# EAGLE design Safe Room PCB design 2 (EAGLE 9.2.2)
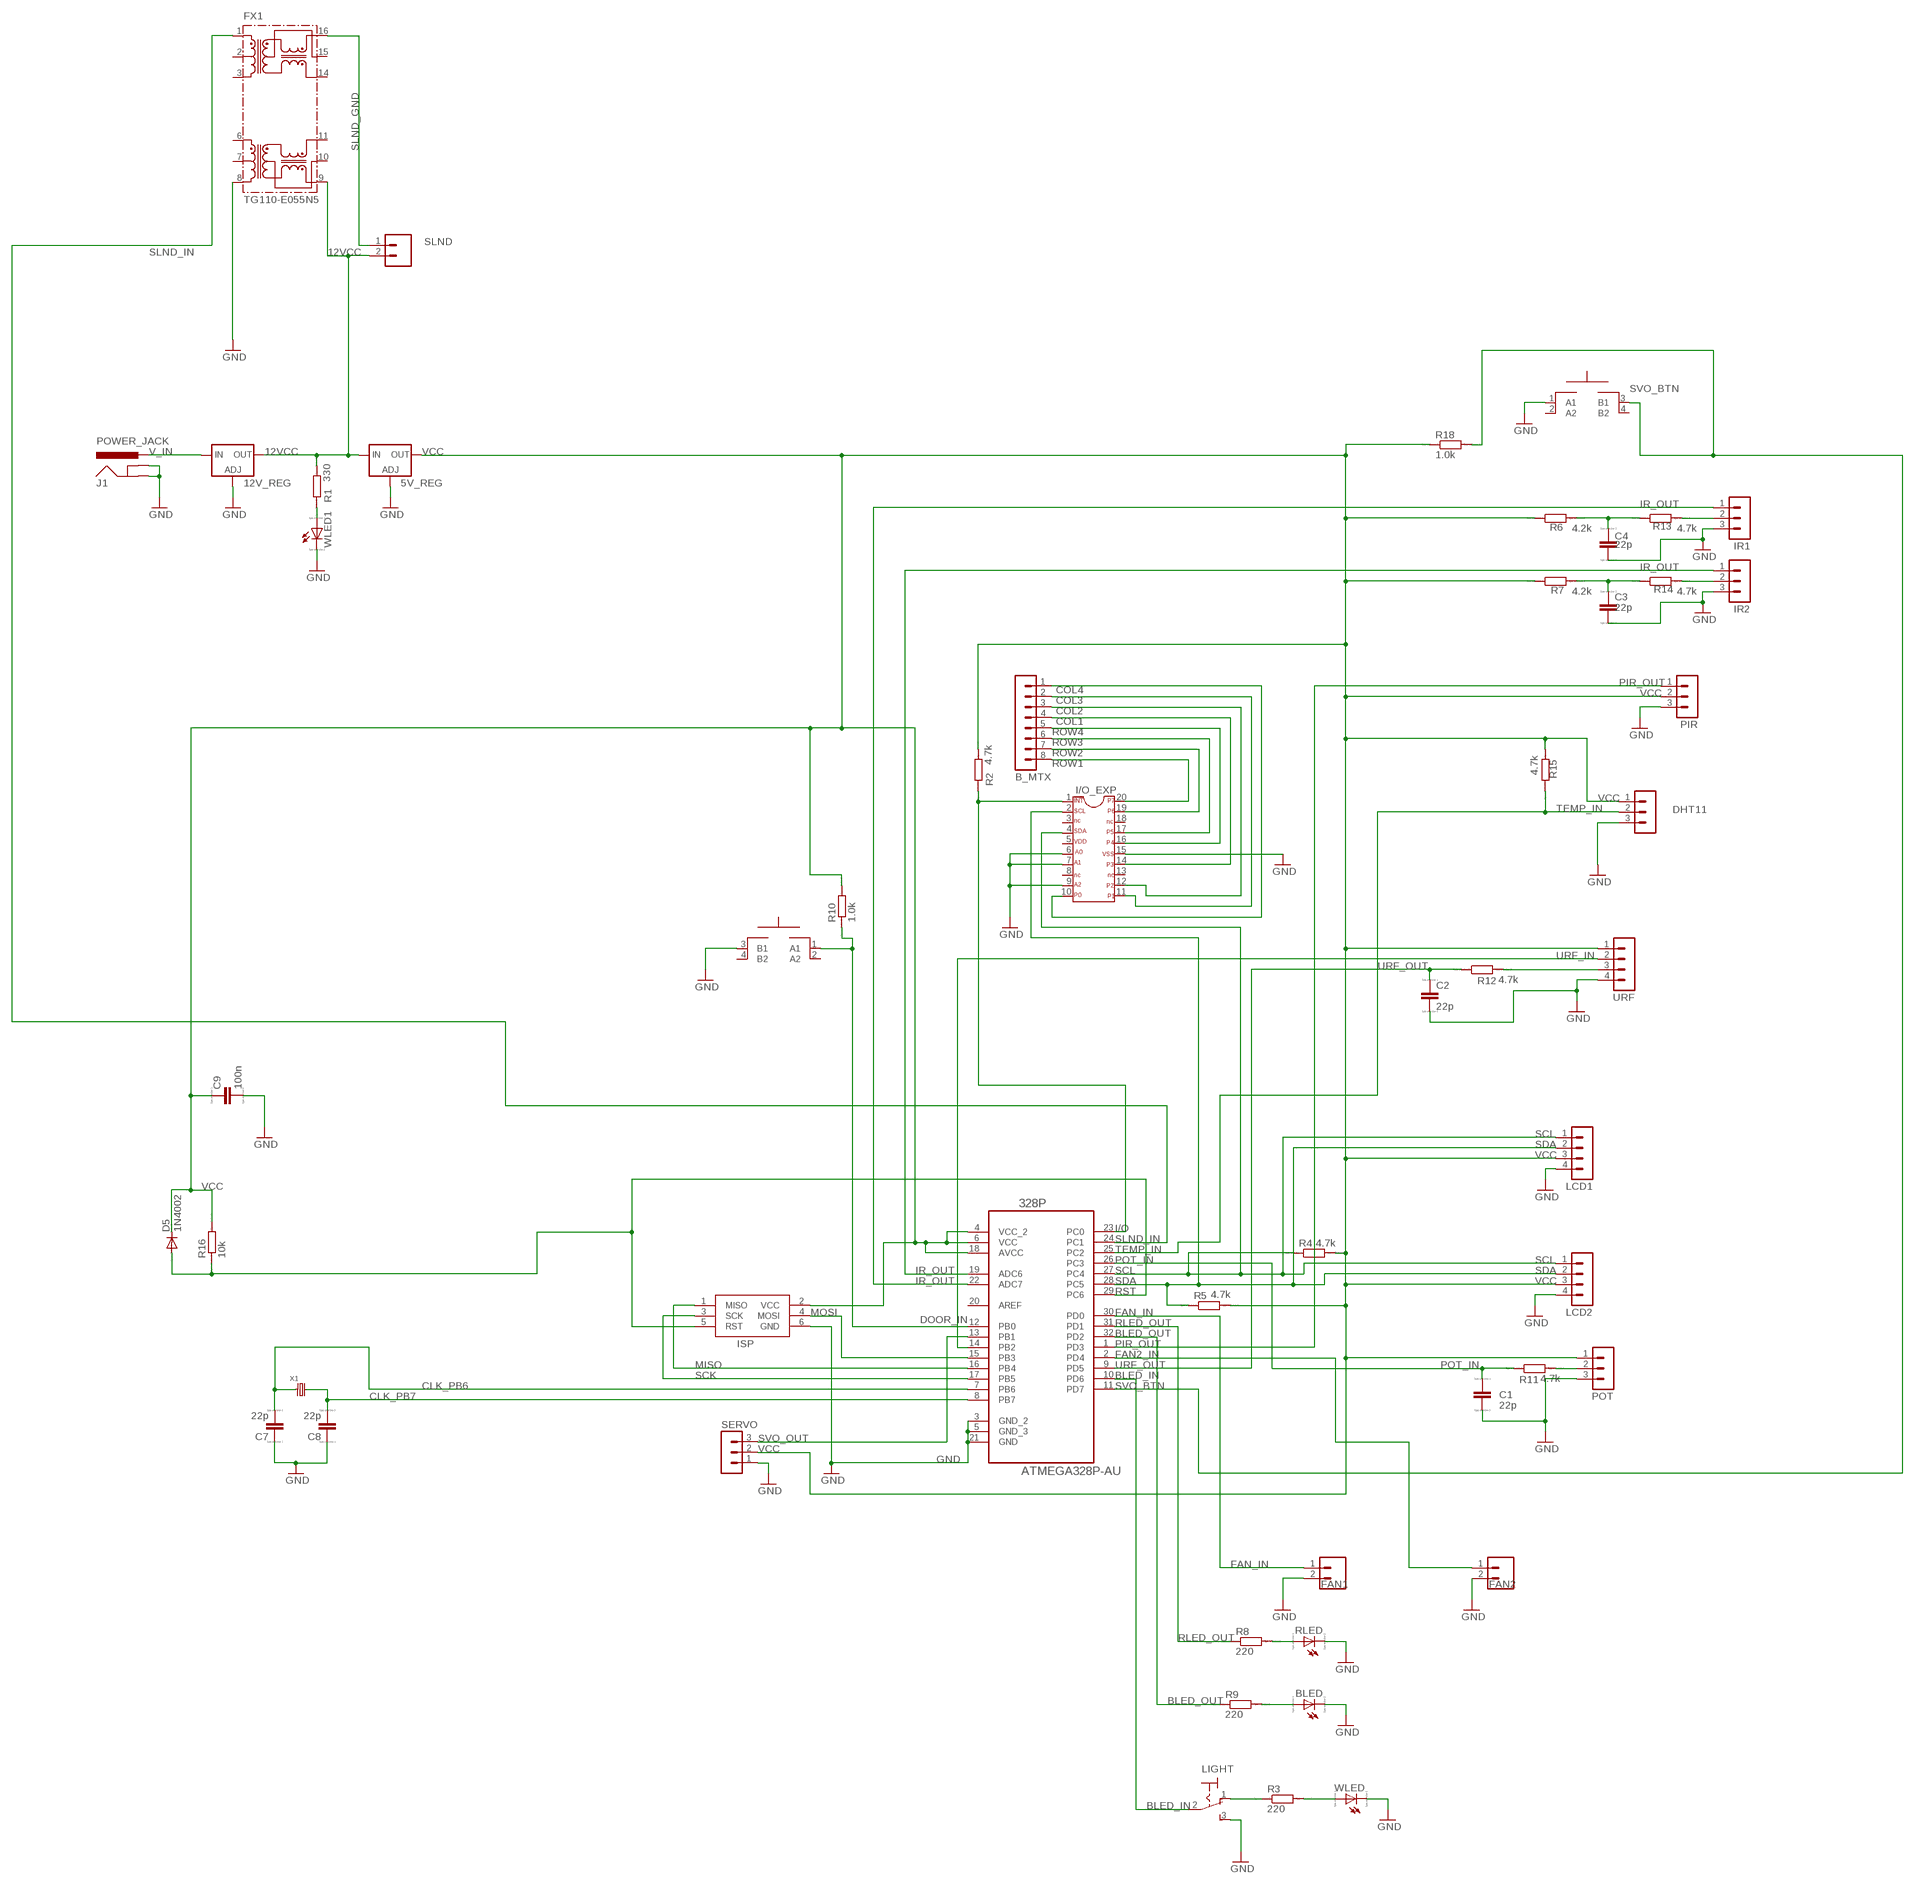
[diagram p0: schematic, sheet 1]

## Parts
5V_REG  LM317MBSTT3  [SOT223]
12V_REG  LD117AV50  [TO220L1]
328P  ATMEGA328P-AU  [QFP80P900X900X120-32N]
B_MTX  MA08-1  [MA08-1]
BLED  LED_E  [LED_1206]
C1  22p  C  [C0805]
C2  22p  C  [C0805]
C3  22p  C  [C0805]
C4  22p  C  [C0805]
C7  22p  C  [C0805]
C8  22p  C  [C0805]
C9  100n  C  [C0805]
D5  1N4002  1N4004  [DO41-10]
DHT11  MA03-1  [MA03-1]
DOOR  MOMENTARYBUTTON  [SPST_NO_SMD]
FAN1  M02  [02P]
FAN2  M02  [02P]
FX1  TG110-E055N5  [N5]
I/O_EXP  PCF8574_20TSSOP  [TSSOP20]
IR1  MA03-1  [MA03-1]
IR2  MA03-1  [MA03-1]
ISP  AVRISP-6  [AVRISP]
J1  POWER_JACK  [POWER_JACK_PTH]
LCD1  MA04-1  [MA04-1]
LCD2  MA04-1  [MA04-1]
LIGHT  320-916  [320-916]
PIR  MA03-1  [MA03-1]
POT  MA03-1  [MA03-1]
R1  330  R  [R0805]
R2  4.7k  R  [R0805]
R3  220  R  [R0805]
R4  4.7k  R  [R0805]
R5  4.7k  R  [R0805]
R6  4.2k  R  [R0805]
R7  4.2k  R  [R0805]
R8  220  R  [R0805]
R9  220  R  [R0805]
R10  1.0k  R  [R0805]
R11  4.7k  R  [R0805]
R12  4.7k  R  [R0805]
R13  4.7k  R  [R0805]
R14  4.7k  R  [R0805]
R15  4.7k  R  [R0805]
R16  10k  R  [R0805]
R18  1.0k  R  [R0805]
RLED  LED_E  [LED_1206]
SERVO  MA03-1  [MA03-1]
SLND  M02  [02P]
SVO_BTN  MOMENTARYBUTTON  [SPST_NO_SMD]
URF  MA04-1  [MA04-1]
WLED  LED_E  [LED_1206]
WLED1  LED_E  [LED_1206]
X1  ECS-80-18-5PX-TR  [HC49/US]

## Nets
12VCC: 5V_REG.3(IN) 12V_REG.2(OUT) FX1.9 R1.2 SLND.2
BLED_IN: 328P.10(PD6) LIGHT.2(P)
BLED_OUT: 328P.32(PD2) R9.1
CLK_PB6: 328P.7(PB6) C7.2 X1.P$1(XIN)
CLK_PB7: 328P.8(PB7) C8.2 X1.P$2(XOUT)
COL1: B_MTX.4 I/O_EXP.14
COL2: B_MTX.3 I/O_EXP.12
COL3: B_MTX.2 I/O_EXP.11
COL4: B_MTX.1 I/O_EXP.10
DOOR_IN: 328P.12(PB0) DOOR.1(A1) R10.1
FAN2_IN: 328P.2(PD4) FAN2.1
FAN_IN: 328P.30(PD0) FAN1.1
GND: 5V_REG.1(ADJ) 12V_REG.1(ADJ) 328P.3(GND_2) 328P.5(GND_3) 328P.21(GND) BLED.C C1.2 C2.2 C3.2 C4.2 C7.1 C8.1 C9.2 DHT11.3 DOOR.3(B1) FAN1.2 FAN2.2 FX1.8 I/O_EXP.6 I/O_EXP.7 I/O_EXP.9 I/O_EXP.15 IR1.3 IR2.3 ISP.6(GND) J1.GND J1.GNDBREAK LCD1.4 LCD2.4 LIGHT.3(S) PIR.3 POT.3 RLED.C SERVO.1 SVO_BTN.1(A1) URF.4 WLED1.C WLED.C
I/O: 328P.23(PC0) I/O_EXP.1 R2.1
IR_OUT: 328P.19(ADC6) 328P.22(ADC7) IR1.1 IR2.1
MISO: 328P.16(PB4) ISP.1(MISO)
MOSI: 328P.15(PB3) ISP.4(MOSI)
N$3: C3.1 R7.2 R14.1
N$4: R8.2 RLED.A
N$5: BLED.A R9.2
N$7: R3.2 WLED.A
N$8: R1.1 WLED1.A
N$9: LIGHT.1(O) R3.1
N$24: POT.2 R11.2
N$25: R12.2 URF.3
N$26: C4.1 R6.2 R13.1
N$27: IR2.2 R14.2
N$28: IR1.2 R13.2
PIR_OUT: 328P.1(PD3) PIR.1
POT_IN: 328P.26(PC3) C1.1 R11.1
RLED_OUT: 328P.31(PD1) R8.1
ROW1: B_MTX.8 I/O_EXP.20
ROW2: B_MTX.7 I/O_EXP.19
ROW3: B_MTX.6 I/O_EXP.17
ROW4: B_MTX.5 I/O_EXP.16
RST: 328P.29(PC6) D5.A ISP.5(RST) R16.1
SCK: 328P.17(PB5) ISP.3(SCK)
SCL: 328P.27(PC4) I/O_EXP.4 LCD1.1 LCD2.1 R4.1
SDA: 328P.28(PC5) I/O_EXP.2 LCD1.2 LCD2.2 R5.1
SLND_GND: FX1.16 SLND.1
SLND_IN: 328P.24(PC1) FX1.1
SVO_BTN: 328P.11(PD7) R18.2 SVO_BTN.3(B1)
SVO_OUT: 328P.13(PB1) SERVO.3
TEMP_IN: 328P.25(PC2) DHT11.2 R15.1
URF_IN: 328P.14(PB2) URF.2
URF_OUT: 328P.9(PD5) C2.1 R12.1
V_IN: 12V_REG.3(IN) J1.PWR
VCC: 5V_REG.4(OUT) 328P.4(VCC_2) 328P.6(VCC) 328P.18(AVCC) C9.1 D5.C DHT11.1 ISP.2(VCC) LCD1.3 LCD2.3 PIR.2 POT.1 R2.2 R4.2 R5.2 R6.1 R7.1 R10.2 R15.2 R16.2 R18.1 SERVO.2 URF.1
Unconnected: 328P.20(AREF) DOOR.2(A2) DOOR.4(B2) FX1.2 FX1.3 FX1.6 FX1.7 FX1.10 FX1.11 FX1.14 FX1.15 I/O_EXP.3 I/O_EXP.5 I/O_EXP.8 I/O_EXP.13 I/O_EXP.18 SVO_BTN.2(A2) SVO_BTN.4(B2)

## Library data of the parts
5V_REG = v-reg:LM317?*: 500 mA Adjustable Output Positive Voltage Regulator Source: http://www.onsemi.co.jp .. LM317M-D.PDF; PARTNUMBER: LM317M
12V_REG = ECE388:LD117A?*: Low drop fixed and adjustable positive voltage regulators 1 A Source: http://www.st.com/stonline/products/literature/ds/7194/ld1117axx.pdf
328P = Atmel_By_element14_Batch_1-00:ATMEGA328P-AU: 8-bit Microcontroller with In-System Programmable Flash; MPN: ATMEGA328P-AU; OC_FARNELL: 1715486; OC_NEWARK: 14R4631; PACKAGE: TQFP-32; SUPPLIER: Atmel
B_MTX = con-lstb:MA08-1: PIN HEADER; OC_FARNELL: unknown; OC_NEWARK: unknown
BLED RLED WLED WLED1 = eagle-ltspice:LED_E: LED; SPICEMODEL: NONE; SPICEPREFIX: D; SPICETYPE: diode
C1-C4 C7-C9 = eagle-ltspice:C: CAPACITOR, European symbol; SPICEMODEL: NONE; SPICEPREFIX: C
D5 = diode:1N4004: DIODE
DHT11 IR1 IR2 PIR POT SERVO = con-lstb:MA03-1: PIN HEADER; OC_FARNELL: unknown; OC_NEWARK: unknown
DOOR SVO_BTN = ECE388:MOMENTARYBUTTON
FAN1 FAN2 SLND = con-amp-quick:M02: AMP QUICK CONNECTOR; OC_FARNELL: unknown; OC_NEWARK: unknown
FX1 = halo-electronics:TG110-E*N5: E-Ultra (TM) 10/100BASE-TX SOIC-16 Fast Ethernet Magnetic Modules Source: www.haloelectronics.com .. e-ultra.pdf
I/O_EXP = MY_LIBRARY:PCF8574_20TSSOP
ISP = ECE388:AVRISP: AVR ISP HEADER Standard 6 pin header for AVR programming
J1 = SparkFun-Connectors:POWER_JACK: Power Jack Connector This is the standard 5.5mm barrel jack for power. The PTH is the most common, proven, reliable, footprint. The Slot footprint only works if the mill layer is transmitted to the PCB fab house so be warned. Here are the connectors we sell at SparkFun: DC Barrel Power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; PROD_ID: CONN-08197
LCD1 LCD2 URF = con-lstb:MA04-1: PIN HEADER; OC_FARNELL: unknown; OC_NEWARK: unknown
LIGHT = switch:320-916: TOGGLE SWITCH distributor RS Components
R1-R16 R18 = eagle-ltspice:R: RESISTOR, European symbol; SPICEMODEL: NONE; SPICEPREFIX: R
X1 = ECE388:ECS-80-18-5PX-TR

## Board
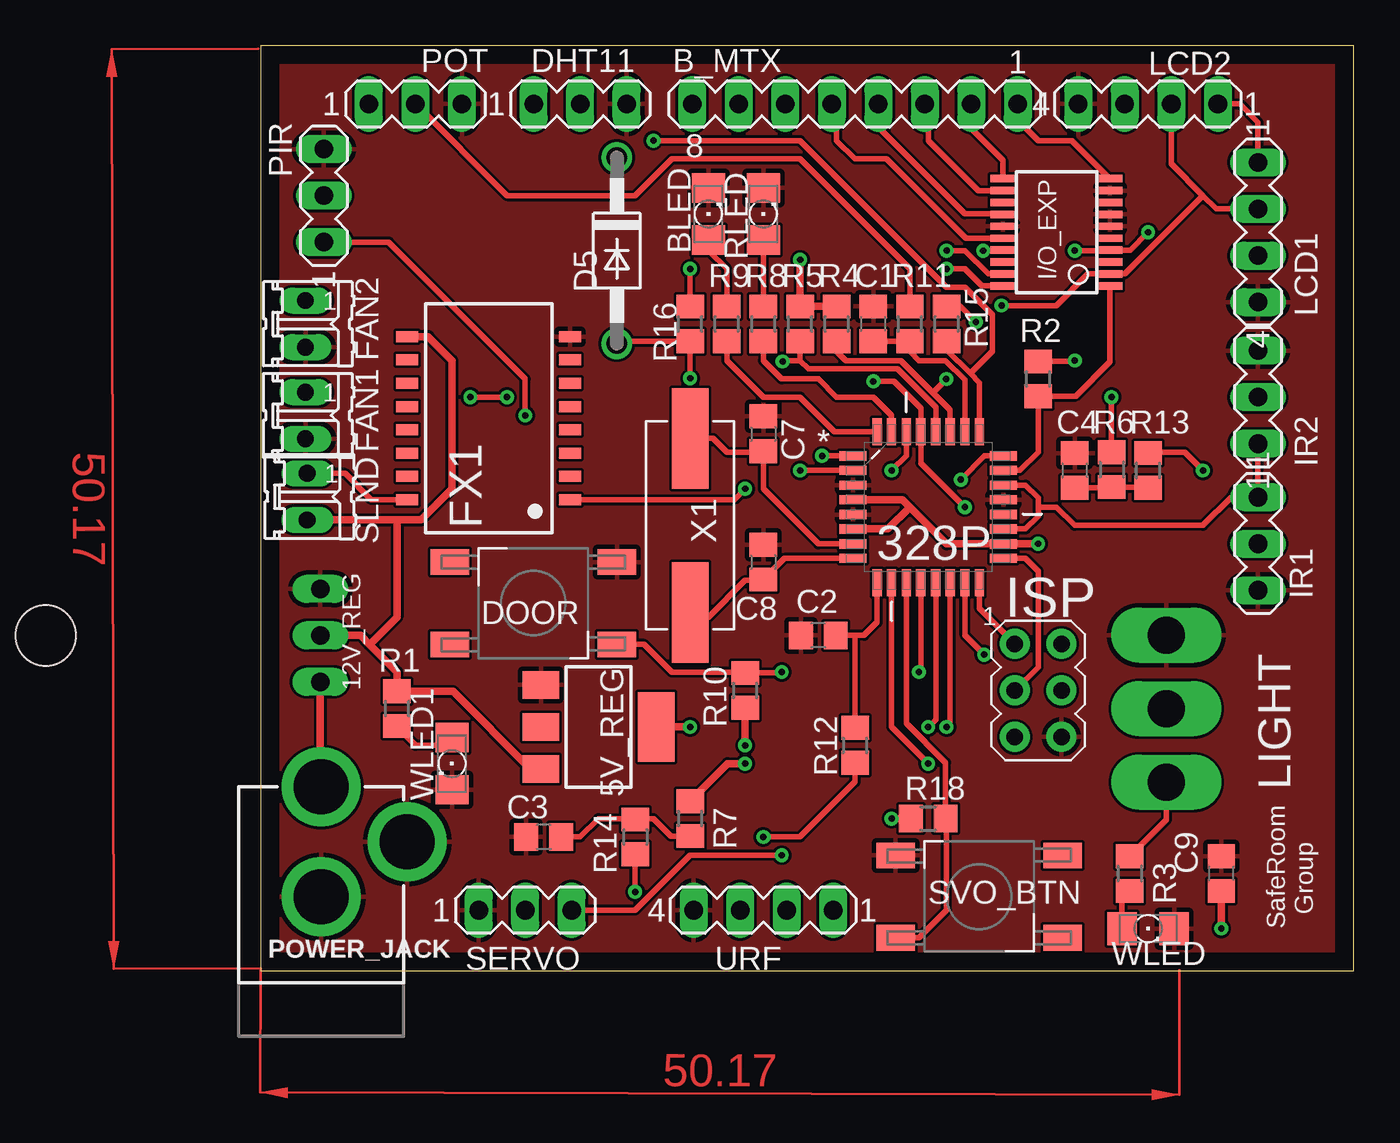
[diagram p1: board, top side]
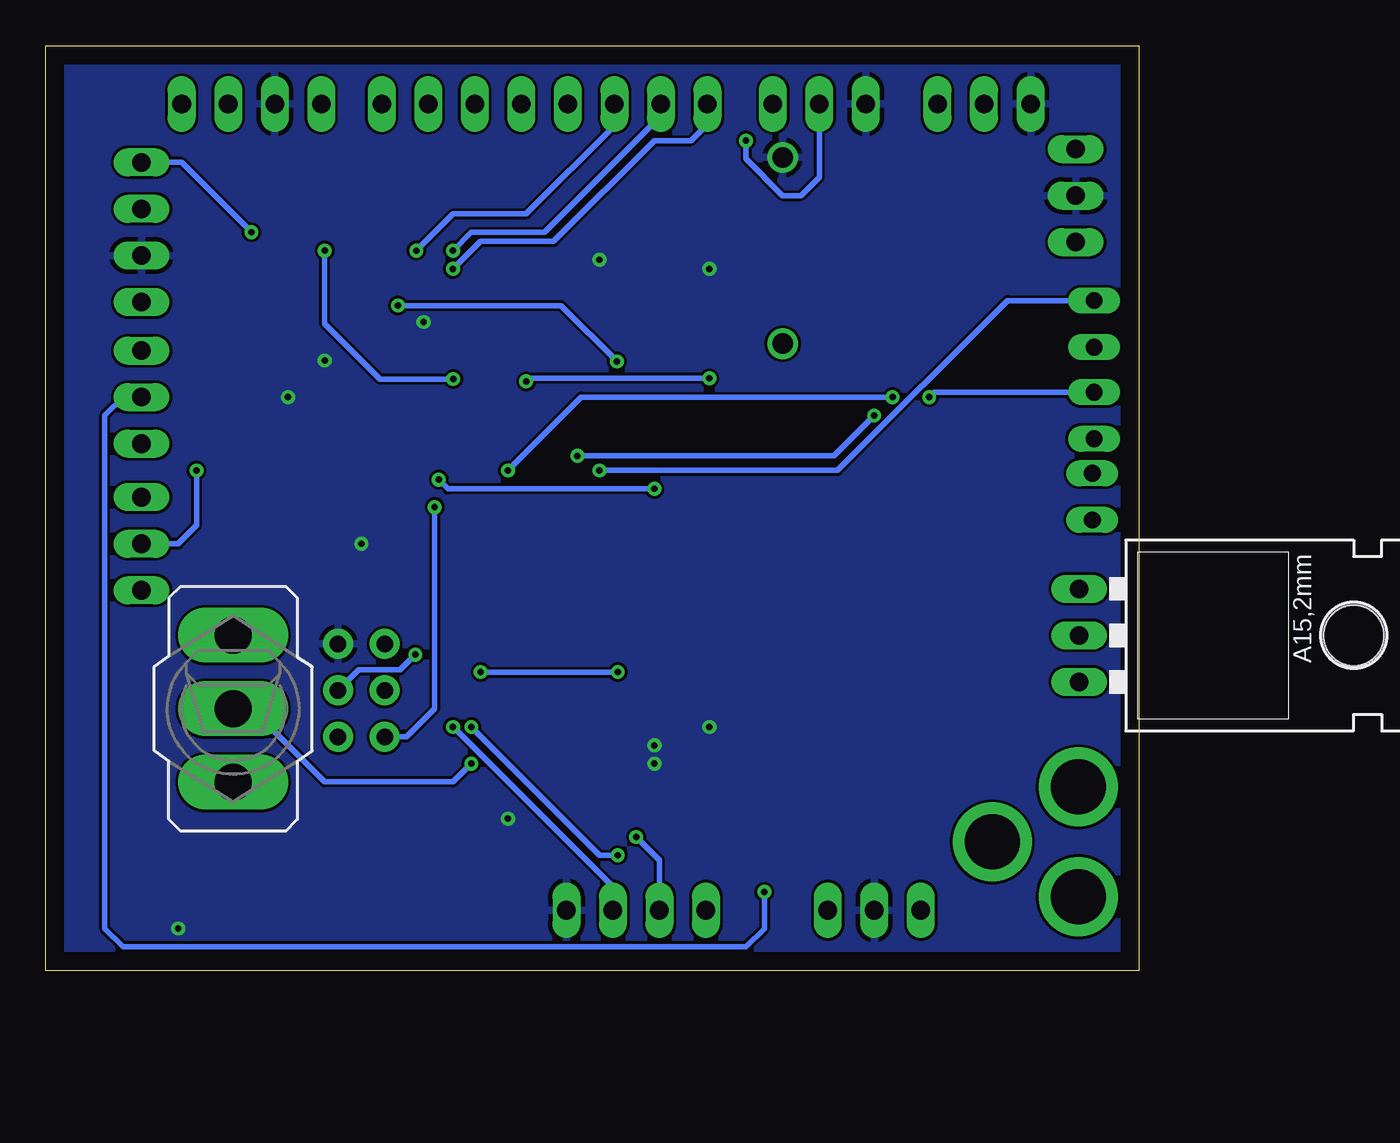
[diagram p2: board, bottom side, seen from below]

Size 59.67 x 50.48 mm. Coordinates in mm from the lower left corner, seen from the top.
Outline: 0,0 59.67,0 59.67,50.48 0,50.48 0,0
Copper layers (1*16): Top 0.035mm / dielectric 1.5mm / Bottom 0.035mm
Design rules "default": minimum track width 6mil, minimum drill 0.35mm, track to track 6mil, track to pad 6mil, pad to pad 6mil, via to via 6mil, smd to smd 6mil, copper to edge 40mil, drill to drill 6mil, minimum pad ring 10mil, minimum via ring 8mil, stop-mask expansion 4mil, vias tented up to drill 0mil, thermal gap 10mil

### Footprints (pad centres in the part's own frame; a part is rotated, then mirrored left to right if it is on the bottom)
SOT223 = smd 1.5 x 2: 1 -2.3,-3.15; 2 0,-3.15; 3 2.3,-3.15 | smd 3.8 x 2: 4 0,3.15
TO220L1 = drill 1.016 long: 1 -2.54,-3.81; 2 0,-3.81; 3 2.54,-3.81 | hole 3.302: 0,11.176
QFP80P900X900X120-32N = smd 1.473 x 0.508: 1 -4.115,2.794; 2 -4.115,2.007; 3 -4.115,1.194; 4 -4.115,0.406; 5 -4.115,-0.406; 6 -4.115,-1.194; 7 -4.115,-2.007; 8 -4.115,-2.794; 17 4.115,-2.794; 18 4.115,-2.007; 19 4.115,-1.194; 20 4.115,-0.406; 21 4.115,0.406; 22 4.115,1.194; 23 4.115,2.007; 24 4.115,2.794 | smd 0.508 x 1.473: 9 -2.794,-4.115; 10 -2.007,-4.115; 11 -1.194,-4.115; 12 -0.406,-4.115; 13 0.406,-4.115; 14 1.194,-4.115; 15 2.007,-4.115; 16 2.794,-4.115; 25 2.794,4.115; 26 2.007,4.115; 27 1.194,4.115; 28 0.406,4.115; 29 -0.406,4.115; 30 -1.194,4.115; 31 -2.007,4.115; 32 -2.794,4.115
MA08-1 = drill 1.016 long: 1 -8.89,0; 2 -6.35,0; 3 -3.81,0; 4 -1.27,0; 5 1.27,0; 6 3.81,0; 7 6.35,0; 8 8.89,0
LED_1206 = smd 1.6 x 1.803: A -1.422,0; C 1.422,0
C0805 = smd 1.3 x 1.5: 1 -0.95,0; 2 0.95,0
DO41-10 = drill 1.118: A 5.08,0; C -5.08,0
MA03-1 = drill 1.016 long: 1 -2.54,0; 2 0,0; 3 2.54,0
SPST_NO_SMD = smd 2.108 x 1.397: 1 0,4.496; 2 9.119,4.496; 3 0,0; 4 9.119,0
02P = drill 0.914 long: 1 -1.27,0; 2 1.27,0
N5 = smd 0.6 x 1.2: 1 -4.445,-4.445; 2 -3.175,-4.445; 3 -1.905,-4.445; 4 -0.635,-4.445; 5 0.635,-4.445; 6 1.905,-4.445; 7 3.175,-4.445; 8 4.445,-4.445; 9 4.445,4.445; 10 3.175,4.445; 11 1.905,4.445; 12 0.635,4.445; 13 -0.635,4.445; 14 -1.905,4.445; 15 -3.175,4.445; 16 -4.445,4.445
TSSOP20 = smd 0.4 x 1.35: 1 -2.925,-2.925; 2 -2.275,-2.925; 3 -1.625,-2.925; 4 -0.975,-2.925; 5 -0.325,-2.925; 6 0.325,-2.925; 7 0.975,-2.925; 8 1.625,-2.925; 9 2.275,-2.925; 10 2.925,-2.925; 11 2.925,2.925; 12 2.275,2.925; 13 1.625,2.925; 14 0.975,2.925; 15 0.325,2.925; 16 -0.325,2.925; 17 -0.975,2.925; 18 -1.625,2.925; 19 -2.275,2.925; 20 -2.925,2.925
AVRISP = drill 0.9 pad 1.626: 1 -1.27,2.54; 2 1.27,2.54; 3 -1.27,0; 4 1.27,0; 5 -1.27,-2.54; 6 1.27,-2.54
POWER_JACK_PTH = drill 2.997 pad 4.318: GND 0,7.7; GNDBREAK 4.7,10.7; PWR 0,13.7
MA04-1 = drill 1.016 long: 1 -3.81,0; 2 -1.27,0; 3 1.27,0; 4 3.81,0
320-916 = drill 2.007 long: 1 0,4.013; 2 0,0; 3 0,-4.013
R0805 = smd 1.3 x 1.5: 1 -0.95,0; 2 0.95,0
HC49/US = smd 5.5 x 2: P$1 -4.75,0; P$2 4.75,0

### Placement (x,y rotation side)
5V_REG  18.44,13.3 270 top
12V_REG  -0.56,18.3 270 bottom
328P  36.44,25.3 0 top
B_MTX  32.44,47.3 180 top
BLED  24.44,41.3 90 top
C1  33.44,35.3 90 top
C2  30.44,18.3 180 top
C3  15.44,7.3 180 top
C4  44.44,27.3 90 top
C7  27.44,29.3 270 top
C8  27.44,22.3 270 top
C9  52.44,5.3 90 top
D5  19.44,39.3 270 top
DHT11  17.44,47.3 0 top
DOOR  19.44,22.3 180 top
FAN1  2.44,30.3 270 top
FAN2  2.44,35.3 270 top
FX1  12.45,30.16 90 top
I/O_EXP  43.44,40.3 90 top
IR1  54.44,23.3 270 top
IR2  54.44,31.3 90 top
ISP  42.44,15.3 0 top
J1  3.3,-3.67 0 top
LCD1  54.44,40.3 270 top
LCD2  48.44,47.3 180 top
LIGHT  49.44,14.3 180 bottom
PIR  3.44,42.3 90 top
POT  8.44,47.3 0 top
R1  7.44,14.3 90 top
R2  42.44,32.3 90 top
R3  47.44,5.3 270 top
R4  31.44,35.3 90 top
R5  29.44,35.3 90 top
R6  46.46,27.35 270 top
R7  23.44,8.3 270 top
R8  27.44,35.3 90 top
R9  25.44,35.3 90 top
R10  26.44,15.3 270 top
R11  35.44,35.3 90 top
R12  32.44,12.3 270 top
R13  48.44,27.3 90 top
R14  20.44,7.3 270 top
R15  37.44,35.3 90 top
R16  23.44,35.3 90 top
R18  36.44,8.3 0 top
RLED  27.44,41.3 90 top
SERVO  14.44,3.3 0 top
SLND  2.54,25.88 270 top
SVO_BTN  34.67,1.8 0 top
URF  27.44,3.3 180 top
WLED  48.44,2.3 0 top
WLED1  10.44,11.3 270 top
X1  23.44,24.3 270 top

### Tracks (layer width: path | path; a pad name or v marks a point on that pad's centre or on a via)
12VCC
  Top 0.406: 5V_REG.3 14.74,11 10.49,15.25 R1.2 7.44,16.3 5.94,17.8 | 12V_REG.2 5.44,18.3 5.94,17.8 | SLND.2 7.44,24.61 | 7.44,24.61 8.75,24.61 10.44,26.3 10.44,33.3 9.14,34.6 FX1.9 | 7.44,24.61 7.44,19.3 5.94,17.8
BLED_IN  (via drill 0.35 pad 0.55)
  Top 0.305: 328P.10 34.44,13.31 v36.44,11.3
  Bottom 0.305: v36.44,11.3 37.44,10.3 44.44,10.3 48.44,14.3 LIGHT.2
BLED_OUT
  Top 0.305: 328P.32 31.33,29.42 29.44,31.3 27.44,31.3 25.44,33.3 R9.1
CLK_PB6
  Top 0.305: 328P.7 32.32,23.3 30.44,23.3 27.44,26.3 27.44,28.3 | 27.44,28.3 C7.2 | X1.P$1 24.69,29.05 25.44,28.3 27.44,28.3
CLK_PB7
  Top 0.305: 328P.8 28.6,22.51 C8.2 27.39,21.3 26.44,21.3 24.44,19.3 23.69,19.3 X1.P$2
COL1
  Top 0.305: I/O_EXP.14 40.49,41.3 38.44,41.3 33.71,46.03 B_MTX.4
COL2
  Top 0.305: B_MTX.3 36.44,47.11 36.44,45.3 39.17,42.58 I/O_EXP.12
COL3
  Top 0.305: B_MTX.2 38.79,45.95 40.52,44.23 I/O_EXP.11
COL4
  Top 0.305: I/O_EXP.10 44.29,45.3 42.44,45.3 41.33,46.41 B_MTX.1
DOOR_IN  (via drill 0.35)
  Top 0.305: 19.95,17.3 DOOR.1 20.94,17.81 22.44,16.3 26.39,16.3 R10.1 28.39,16.25 v28.44,16.3 | 328P.12 36.04,16.41 v35.93,16.3
  Bottom 0.305: v35.93,16.3 v28.44,16.3
FAN2_IN  (via drill 0.35)
  Top 0.305: 328P.2 32.32,27.3 v29.44,27.3
  Bottom 0.305: v29.44,27.3 16.44,27.3 7.17,36.57 FAN2.1
FAN_IN  (via drill 0.35)
  Top 0.305: 35.36,29.52 328P.30 35.25,28.11 v34.44,27.3 | v13.44,31.3 v11.44,31.3
  Bottom 0.305: v34.44,27.3 30.44,31.3 v13.44,31.3 | v11.44,31.3 11.17,31.57 FAN1.1
GND
  pour Top: -8,57.24 -8,0 59.19,0 59.19,57.24
I/O
  Top 0.305: 328P.23 40.57,27.3 41.44,27.3 42.44,28.3 42.44,31.25 42.39,31.3 R2.1 44.49,31.35 46.37,33.23 I/O_EXP.1
IR_OUT
  Top 0.305: 328P.22 41.75,26.5 42.44,25.8 42.44,25.3 | 42.44,25.3 42.44,24.8 41.75,24.11 328P.19 | 42.44,25.3 43.44,25.3 44.44,24.3 51.44,24.3 52.98,25.84 IR1.1 IR2.1
MISO
  Top 0.305: ISP.1 39.24,19.78 328P.16
MOSI  (via drill 0.35 pad 0.55)
  Top 0.305: v39.5,17.25 38.45,18.3 328P.15
  Bottom 0.305: ISP.4 42.6,16.42 40.33,16.42 v39.5,17.25
N$3
  Top 0.305: 23.43,7.34 R7.2 22.39,7.35 21.44,8.3 20.49,8.3 R14.1 20.39,8.3 18.44,8.3 17.44,7.3 C3.1
N$4
  Top 0.305: R8.2 RLED.A
N$5
  Top 0.305: BLED.A 24.44,39.3 | 24.44,39.3 24.44,39.25 | R9.2 25.44,38.3 24.44,39.3
N$7
  Top 0.305: R3.2 47.02,3.93 WLED.A
N$8
  Top 0.305: WLED1.A 10.02,12.3 8.44,12.3 7.44,13.3 R1.1
N$9
  Top 0.305: LIGHT.1 49.44,8.25 R3.1
N$24
  Top 0.305: POT.2 13.44,42.3 20.44,42.3 22.44,44.3 29.44,44.3 35.44,38.3 R11.2
N$25  (via drill 0.35)
  Top 0.305: R12.2 32.44,10.3 29.44,7.3 v27.44,7.3
  Bottom 0.305: URF.3 26.17,6.03 v27.44,7.3
N$26
  Top 0.305: C4.1 46.42,26.35 R6.2 48.4,26.4 R13.1
N$27  (via drill 0.35)
  Top 0.305: v20.44,4.3 R14.2
  Bottom 0.305: v20.44,4.3 20.44,2.3 21.44,1.3 55.44,1.3 56.44,2.3 56.44,30.3 55.44,31.3 IR2.2
N$28  (via drill 0.35)
  Top 0.305: v51.44,27.3 50.44,28.3 48.49,28.3 R13.2
  Bottom 0.305: IR1.2 52.44,23.3 51.44,24.3 v51.44,27.3
PIR_OUT  (via drill 0.35)
  Top 0.305: 328P.1 v30.65,28.1 | v14.44,30.3 14.44,32.3 6.98,39.76 PIR.1
  Bottom 0.305: v30.65,28.1 16.65,28.1 v14.44,30.3
POT_IN
  Top 0.305: 328P.26 38.44,32.24 37.39,33.3 35.94,33.3 35.44,33.8 R11.1 C1.1
RLED_OUT
  Top 0.305: 27.49,34.3 R8.1 27.44,33.3 28.44,32.3 30.44,32.3 31.44,31.3 33.44,31.3 34.44,30.3 328P.31
ROW1  (via drill 0.35)
  Top 0.305: v37.44,38.3 38.44,38.3 39.37,37.38 I/O_EXP.20
  Bottom 0.305: B_MTX.8 23.55,46.19 24.44,45.3 26.44,45.3 31.94,39.8 35.94,39.8 | v37.44,38.3 35.94,39.8 | 35.94,39.8 35.93,39.82
ROW2  (via drill 0.35)
  Top 0.305: I/O_EXP.19 39.72,38.03 38.44,39.3 v37.44,39.3
  Bottom 0.305: v37.44,39.3 36.44,40.3 32.44,40.3 26.09,46.65 B_MTX.7
ROW3  (via drill 0.35)
  Top 0.305: I/O_EXP.17 40.49,39.3 v39.44,39.3
  Bottom 0.305: v39.44,39.3 37.44,41.3 33.44,41.3 28.63,46.11 B_MTX.6
ROW4
  Top 0.305: I/O_EXP.16 38.5,39.98 34.17,44.3 32.44,44.3 31.44,45.3 31.44,47.03 B_MTX.5
RST  (via drill 0.35, 0.35 pad 0.55)
  Top 0.305: v38.44,25.3 36.04,27.71 328P.29 36.04,30.71 34.58,32.16 v33.44,32.16 | D5.A 19.57,34.35 R16.1 v23.44,32.33
  Bottom 0.305: ISP.5 39.98,12.76 38.44,14.3 v38.44,25.3 | v23.44,32.33 33.27,32.33 v33.44,32.16
SCK
  Top 0.305: 328P.17 41.74,22.51 42.44,21.8 42.44,16.57 ISP.3
SCL  (via drill 0.35)
  Top 0.305: 328P.27 37.64,30.61 36.69,31.55 | R4.1 31.44,33.8 31.94,33.3 34.94,33.3 36.69,31.55 | LCD2.1 53.44,47.3 54.44,46.3 LCD1.1 | v48.44,40.3 47.47,39.33 I/O_EXP.4 46.34,39.3 v44.44,39.3 | 36.69,31.55 v37.43,32.29
  Bottom 0.305: v48.44,40.3 52.25,44.11 LCD1.1 | v37.43,32.29 41.43,32.29 44.44,35.3 v44.44,39.3
SDA  (via drill 0.35)
  Top 0.305: 328P.28 36.85,30.75 34.76,32.85 29.9,32.85 29.44,33.3 | 29.44,33.3 R5.1 | LCD1.2 52.17,41.57 51.44,42.3 | LCD2.2 49.71,44.03 51.44,42.3 | 51.44,42.3 47.17,38.03 I/O_EXP.2 45.17,38.03 43.44,36.3 v40.44,36.3 | 29.44,33.3 28.54,33.3 v28.49,33.25
  Bottom 0.305: v28.49,33.25 31.54,36.3 v40.44,36.3
SLND_GND
  Top 0.305: FX1.16 6.03,25.71 4.6,27.14 SLND.1
SLND_IN  (via drill 0.35)
  Top 0.305: 328P.24 39.52,28.1 v38.22,26.8 | FX1.1 25.85,25.71 v26.44,26.3
  Bottom 0.305: v38.22,26.8 37.72,26.3 v26.44,26.3
SVO_BTN
  Top 0.305: 328P.11 35.25,13.5 37.39,11.35 R18.2 37.44,8.25 37.44,3.3 35.94,1.8 SVO_BTN.3
SVO_OUT  (via drill 0.35)
  Top 0.305: 328P.13 36.85,13.71 v36.44,13.3 | v28.44,6.3 23.44,6.3 20.44,3.3 SERVO.3
  Bottom 0.305: v36.44,13.3 29.44,6.3 v28.44,6.3
TEMP_IN  (via drill 0.35)
  Top 0.305: 328P.25 39.24,32.1 38.74,32.6 | R15.1 37.44,33.89 38.74,32.6 | 38.74,32.6 39.94,33.8 39.94,35.8 38.44,37.3 37.44,37.3 29.44,45.3 v21.44,45.3
  Bottom 0.305: v21.44,45.3 21.44,44.3 19.44,42.3 18.44,42.3 17.44,43.3 DHT11.2
URF_IN  (via drill 0.35)
  Top 0.305: v37.44,13.3 37.64,13.5 328P.14
  Bottom 0.305: URF.2 28.71,4.57 v37.44,13.3
URF_OUT
  Top 0.305: 328P.9 33.65,19.01 32.94,18.3 32.44,18.3 | 32.44,18.3 C2.1 | R12.1 32.44,18.3
V_IN
  Top 0.406: 12V_REG.3 3.25,10.08
  Top 0.508: 3.25,10.08 J1.PWR
VCC  (via drill 0.35)
  Top 0.305: R16.2 v23.44,38.3 | R2.2 44.39,33.25 v44.44,33.3 | R6.1 46.44,28.32 v46.44,31.3 | R15.2 38.19,36.25 v39.04,35.4
  Top 0.406: 328P.6 34.25,24.11 35.44,25.3 | 328P.4 35.04,25.71 35.44,25.3 | 35.44,25.3 37.44,23.3 328P.18 40.57,23.3 v42.44,23.3 | R10.2 v26.44,12.3 | 5V_REG.4 v23.44,13.3 | R7.1 25.49,11.3 v26.44,11.3 | R18.1 v34.44,8.3 | R4.2 R5.2 v29.44,38.8 | C9.1 v52.44,2.3
  pour Bottom: -12.56,53.3 59.44,53.3 59.44,0.3 -12.56,0.3
(copper drawn outside any net)
  shapes: Top area x2

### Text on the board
tPlace: SafeRoom / Group

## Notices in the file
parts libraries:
SparkFun-Connectors: Licensing: Creative Commons ShareAlike 4.0 International - https://creativecommons.org/licenses/by-sa/4.0
